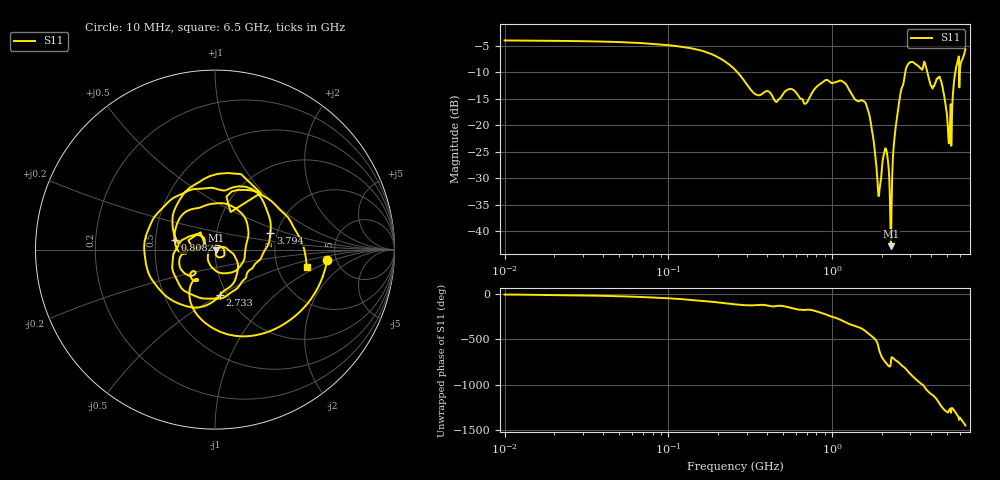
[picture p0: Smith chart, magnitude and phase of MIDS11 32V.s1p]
!Keysight Technologies,E5080B,MY59100498,A.17.05.10
!Date: Wednesday, August 30, 2023 14:19:15
!Correction: S11(C  1-Port  )
!S1P File: Measurement: S11:Log Frequency Sweep
# Hz S  dB  R 50
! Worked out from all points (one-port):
!   1601 points, 10 MHz to 6.5 GHz, reference 50 ohm
!   lowest |S11| = -42.9 dB at 2.278 GHz (marker M1), VSWR 1.01, Z = 50.6 - j0.468 ohm
!   |S11| at or under -10 dB: 263.2 MHz to 2.792 GHz (2.529 GHz wide, 166 % of centre); 3.804 GHz to 5.643 GHz (1.839 GHz wide, 38.9 % of centre); 5.956 GHz to 6.005 GHz (48.45 MHz wide, 0.81 % of centre)
!   S11 on the Smith chart (normalised r, x): 10 MHz: 4.21, -0.79; 808.2 MHz: 0.63, +0.07; 2.733 GHz: 0.92, -0.50; 3.794 GHz: 1.84, +0.38; 6.5 GHz: 2.94, -0.77
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1e7  -4.04 -5.2
2.256172e7  -4.13 -11.2
5.069748e7  -4.35 -24.4
1.139202e8  -5.13 -53.0
2.54951e8  -9.55 -113.4
3.467928e8  -14.32 -122.0
5.728895e8  -13.29 -156.1
6.873597e8  -15.96 -173.1
8.081777e8  -12.71 166.8
1.081653e9  -11.77 88.6
1.292537e9  -13.76 24.6
1.641229e9  -16.85 -66.5
1.92971e9  -33.23 110.8
2.135226e9  -24.62 -41.0
2.278101e9  -42.85 -40.0
2.450294e9  -19.96 -11.6
2.733293e9  -11.84 -83.9
2.904406e9  -8.50 -135.5
3.098749e9  -8.09 172.0
3.360066e9  -8.87 114.5
3.584899e9  -9.11 76.4
3.793935e9  -9.86 16.6
4.371419e9  -11.28 -88.4
4.645083e9  -11.98 -160.6
5.202588e9  -21.86 166.7
5.618531e9  -10.34 140.3
5.946149e9  -7.84 51.0
6.5e9  -5.69 -10.6
